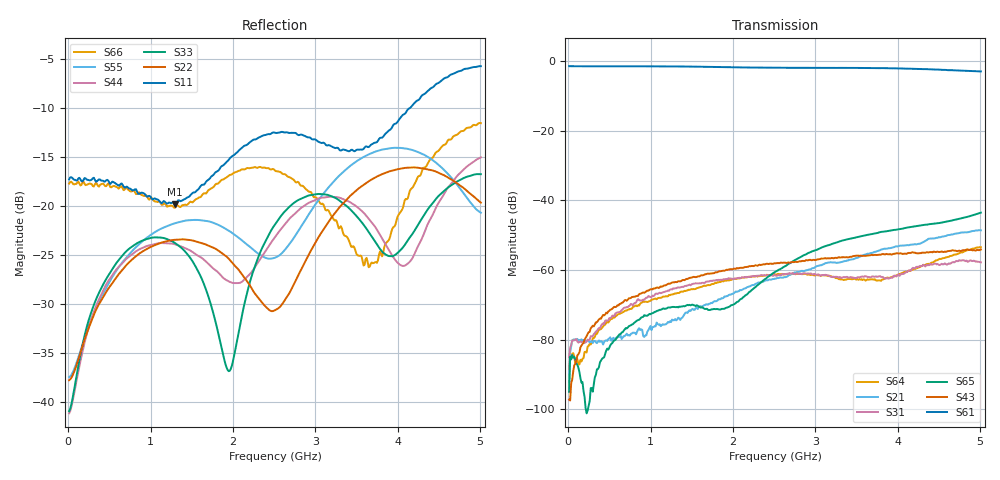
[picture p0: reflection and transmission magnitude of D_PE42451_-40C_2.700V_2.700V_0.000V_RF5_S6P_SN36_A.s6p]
! Device ID: PE42451
! Serial: 36
! Insertion: A
! Temp: -40C
! VDD: 2.700
! Control_Hi: 100.000
! Control_Lo: 0.000
! Logic State: RF5
! Port 1: RFC
! Port 2: RF1
! Port 3: RF2
! Port 4: RF3
! Port 5: RF4
! Port 6: RF5
! V1 = 2.70
! V2 = 0.00
! V3 = 2.70
! V4 = 0.00
! IDD: 1.072140e-05
#  Hz  S  RI  R  50
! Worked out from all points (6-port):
!   401 points, 10 MHz to 5.01 GHz, reference 50 ohm
!   strongest paths, dB at 10 MHz, 1.26 GHz, 2.51 GHz, 3.76 GHz, 5.01 GHz:
!     S61: -1.4, -1.5, -1.8, -1.9, -2.9
!     S43: -97.2, -63.6, -58.1, -55.6, -54.1
!     S65: -95.0, -70.6, -60.5, -49.3, -43.5
!     S31: -85.0, -65.6, -61.5, -61.9, -57.8
!     S21: -92.3, -74.2, -62.4, -54.5, -48.6
!     S64: -88.4, -67.0, -61.2, -63.0, -53.4
!   lowest |S11| = -19.8 dB at 1.298 GHz (marker M1), VSWR 1.23, Z = 54.2 - j9.83 ohm
!   |S11| at or under -10 dB: start of sweep to 4.149 GHz
